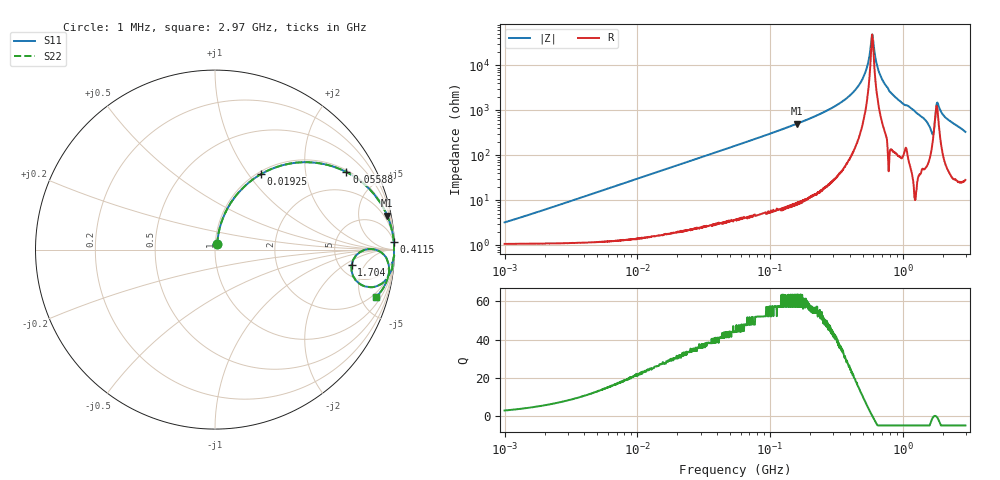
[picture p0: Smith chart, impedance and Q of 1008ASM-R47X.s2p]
!s-Parameter Generated by FASTRON Sdn. Bhd.
!FASTRON P/N : 1008ASM-R47X
!Keysight Technologies: E4991B_MY54100416_A.01.15
!Date: Tue Nov 21 09:18:49 2023
!Version  :Rev00  Wed Nov 22 15:15:29 2023
!Data & Calibration Information:
!Freq  S11  S21  S12  S22
!PortZ  Port1:50+j0  Port2:50+j0
!When reading reference impedance value at option line is always used.
! Remarks : This data is being provided solely for informational purposes.
# Hz S dB R 50
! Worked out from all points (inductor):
!   1599 points, 1 MHz to 2.97 GHz, reference 50 ohm
!   read as one part in series: L = 484 nH near 1.062 MHz
!   highest Q = 63.5 at 160.6 MHz (marker M1), where L = 503 nH
!   self-resonance near 590 MHz
!   S11 on the Smith chart (normalised r, x): 1 MHz: 1.02, +0.06; 19.25 MHz: 1.04, +1.15; 55.88 MHz: 1.07, +3.34; 411.5 MHz: 3, +46; 1.704 GHz: 6.37, -2.70; 2.97 GHz: 1.57, -6.62
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1000000  -29.90 68.9  -0.10 -1.7  -0.10 -1.7  -29.90 68.9
3804036  -18.90 77.9  -0.15 -6.5  -0.15 -6.5  -18.90 77.9
1.439846e7  -8.12 64.7  -0.87 -23.1  -0.87 -23.1  -8.12 64.7
1.924694e7  -6.14 58.6  -1.37 -29.5  -1.37 -29.5  -6.14 58.6
5.477226e7  -1.46 31.1  -5.74 -57.6  -5.74 -57.6  -1.46 31.1
5.587962e7  -1.41 30.6  -5.87 -58.2  -5.87 -58.2  -1.41 30.6
1.606197e8  -0.19 11.1  -14.30 -78.0  -14.30 -78.0  -0.19 11.1
2.073156e8  -0.11 8.2  -16.90 -80.8  -16.90 -80.8  -0.11 8.2
4.114912e8  -0.02 2.5  -27.40 -85.0  -27.40 -85.0  -0.02 2.5
5.128394e8  -0.02 0.9  -35.60 -82.4  -35.60 -82.4  -0.02 0.9
5.418594e8  -0.02 0.6  -39.80 -78.3  -39.80 -78.3  -0.02 0.6
5.753936e8  -0.02 0.2  -48.90 -55.7  -48.90 -55.7  -0.02 0.2
5.899715e8  -0.02 0.0  -53.80 -1.4  -53.80 -1.4  -0.02 0.0
6.652545e8  -0.02 -0.8  -36.90 80.5  -36.90 80.5  -0.02 -0.8
7.846996e8  -0.01 -2.0  -29.10 87.1  -29.10 87.1  -0.01 -2.0
1.466741e9  -0.21 -8.9  -16.20 76.5  -16.20 76.5  -0.21 -8.9
1.645649e9  -1.14 -13.7  -11.80 54.5  -11.80 54.5  -1.14 -13.7
1.704314e9  -2.32 -6.6  -11.90 20.1  -11.90 20.1  -2.32 -6.6
1.791767e9  -0.65 -1.1  -22.60 13.2  -22.60 13.2  -0.65 -1.1
1.846379e9  -0.35 -3.3  -23.20 53.0  -23.20 53.0  -0.35 -3.3
2.124078e9  -0.20 -8.3  -16.80 76.8  -16.80 76.8  -0.20 -8.3
2.970126e9  -0.58 -16.3  -11.00 68.8  -11.00 68.8  -0.58 -16.3
